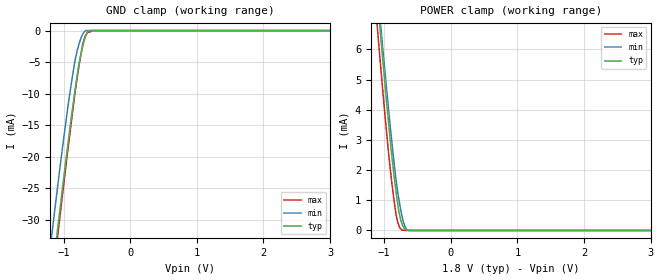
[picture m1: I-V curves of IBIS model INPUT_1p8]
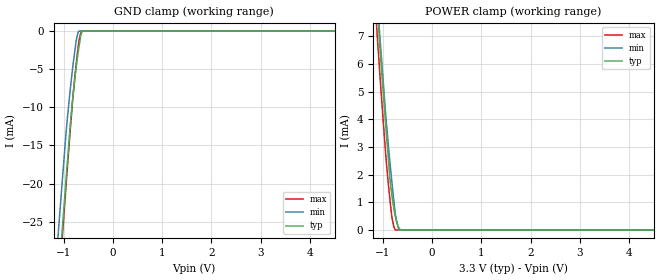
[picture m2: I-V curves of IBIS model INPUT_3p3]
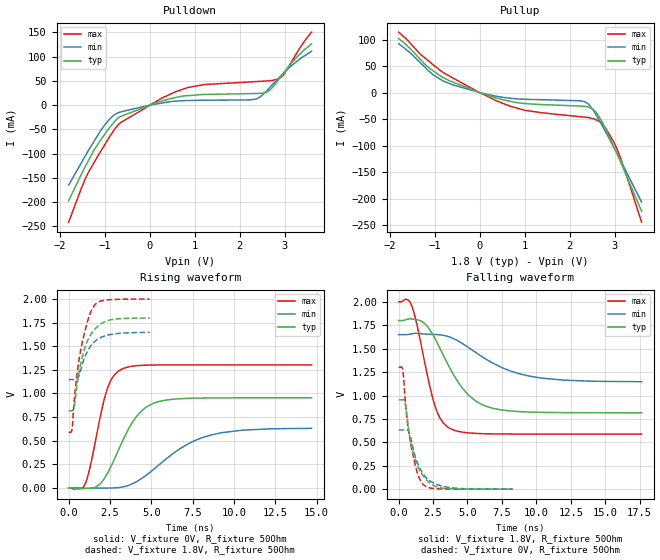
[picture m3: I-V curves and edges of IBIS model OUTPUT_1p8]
|Texas Instruments Incorporated
|12-Bit, Nanopower, 4-Wire
|   Micro TOUCH SCREEN CONTROLLER with I2C Interface
| Marketing part#   Digital Voltage Range   Package-type   #pins
|TSC2017IYZGT   1.6V - 3.6V   3X4 Array, WCSP   12-pins
|TSC2017IYZGR   1.6V - 3.6V   3X4 Array, WCSP   12-pins
[IBIS Ver]   4.0
[File name]   tsc2017.ibs
|SIMDE Ver   V2.0 - 201002 - RHL4 - Build 372
[File Rev]   1.0
[Date]   02/18/2011
[Source]   Texas Instruments Incorporated.
   Analog-eLab, HPA
   12500 TI Blvd
   Dallas, TX -75243
   For Support e-mail: elab_ibis@list.ti.com
[Notes]   Revision History:
   1.0: 02/18/2011
   - Initial version of the model
   - Model generated from simulations in TISPICE
   - Model matched to SPICE simulation
   - C_comp although listed in numerical order of value are
   obtained from varying PVT conditions. For PVT conditions for
   each specific value refer the buffer description under
   respective [Model]. IBIS model user is responsible for using
   appropriate C_comp to simulate for Signal Integrity.
   1.1: 03/17/2011
   - Removed 50 ohm loads rising waveform and falling waveform data
   for I2C_fast_mode_1p8, I2C_fast_mode_3p3,
   I2C_high_mode_1p8, and I2C_high_mode_3p3 buffers.
[Disclaimer]
 This product is designed as an aid for customers of Texas Instruments.
 No warranties, either expressed or implied, with respect to this third
 party software (if any) or with respect to its fitness for any
 particular purpose is claimed by Texas Instruments or the author. The
 software (if any) is provided solely on an "as is" basis. The entire
 risk as to its quality and performance is with the customer
[Copyright] (C) Copyright 2011 Texas Instruments Incorporated.
   All rights reserved.
|   TSC2017
[Component]   tsc2017yzg
[Manufacturer] TI
[Package]   |12 WCSP -  YZG package
| variable   typ   min   max
R_pkg   5.30000E-02   1.00000E-03   1.81000E-01
L_pkg   5.36400E-01nH 1.07000E-01nH 1.65500E+00nH
C_pkg   7.09400E-01pF 4.30000E-01pF 1.27400E+00pF
[Pin] signal_name  model_name  R_pin  L_pin C_pin
A1   AUX   TERM   0.007   0.211nH   0.551pF
A2   VDD_REF   POWER   0.004   0.165nH   0.711pF
A3   XP   TERM   0.011   0.249nH   0.568pF
B1   _PINTDAV   OUTPUT   0.181   1.655nH   1.274pF
B2   A0   INPUT   0.042   0.651nH   0.989pF
B3   YP   TERM   0.005   0.189nH   0.554pF
C1   SDA   I2C   0.001   0.107nH   0.430pF
C2   _RESET   INPUT   0.101   0.728nH   0.719pF
C3   XN   TERM   0.007   0.190nH   0.517pF
D1   SCL   I2C   0.163   1.109nH   0.887pF
D2   GND   GND   0.010   0.142nH   0.687pF
D3   YN   TERM   0.012   0.275nH   0.605pF
|   Model Selectors
[Model Selector] INPUT
INPUT_1p8   1.8V digital input
INPUT_3p3   3.3V digital input
|NOTES   Model INPUT split into two Models INPUT_1p6, INPUT_1p8 and
|   INPUT_3p3 to accomodate voltage range of 1.6 V - 3.6V
|   INPUT_1p8 operates in voltage range of 1.65 - 1.8 - 2.0
|   INPUT_3p3 operates in voltage range of 3.0 - 3.3 - 3.6
|   The min pin frequency for Model INPUT is 400 KHz
|   This is referenced with datasheet
[Model Selector] I2C
I2C_fast_mode_1p8   1.8V digital open drain io
I2C_fast_mode_3p3   3.3V digital open drain io
I2C_high_mode_1p8   1.8V digital open drain io
I2C_high_mode_3p3   3.3V digital open drain io
|NOTES   Model I2C split into four Models
|   I2C_fast_mode_1p8, I2C_fast_mode_3p3,
|   I2C_high_mode_1p8 and I2C_high_mode_3p3 to accomodate
|   voltage range of 1.6 V - 3.6V and high speed and fast speed
|   modes. I2C_fast_mode operates at 400 KHz and I2C_high_mode
|   operates at 3.4 MHz. This is referenced with datasheet
[Model Selector] OUTPUT
OUTPUT_1p8   1.8V digital output
OUTPUT_3p3   3.3V digital output
|NOTES   Model OUTPUT split into two Models OUTPUT_1p8 and
|   OUTPUT_3p3 to accomodate voltage range of 1.6 V - 3.6V
|   OUTPUT_1p8 operates in voltage range of 1.65 - 1.8 - 2.0
|   OUTPUT_3p3 operates in voltage range of 3.0 - 3.3 - 3.6
|   The min pin frequency for Model OUTPUT is 400 KHz
|   This is referenced with datasheet
[Model Selector] TERM
TERM_1p8  1.8V nominal termination
TERM_3p3  3.3V nominal termination
|   TERM Models
[Model] TERM_1p8
Model_type Terminator
C_comp   1.0e-20F  1.0e-20F  1.0e-20F
|   typ   min   max
[Voltage Range]   1.8V   1.65V   2.0V
[POWER Clamp Reference]   1.8V   1.65V   2.0V
[GND Clamp Reference]   0V   0V   0V
|Ambient Temperature   25   85   -40
|Junction Temperature
[Temperature Range]   25   85   -40
[Model] TERM_3p3
Model_type Terminator
C_comp   1.0e-20F  1.0e-20F  1.0e-20F
|   typ   min   max
[Voltage Range]   3.3V   3.0V   3.6V
[POWER Clamp Reference]   3.3V   3.0V   3.6V
[GND Clamp Reference]   0V   0V   0V
|Ambient Temperature   25   85   -40
|Junction Temperature
[Temperature Range]   25   85   -40
| Models and submodels in the file (10): INPUT_1p8 (Input), INPUT_3p3 (Input), OUTPUT_1p8 (Output), OUTPUT_3p3 (Output), I2C_fast_mode_1p8 (I/O_open_drain), I2C_fast_mode_3p3 (I/O_open_drain), I2C_high_mode_1p8 (I/O_open_drain), I2C_high_mode_3p3 (I/O_open_drain), TERM_1p8 (Terminator), TERM_3p3 (Terminator)
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|   input_1p8 Model
[Model]   INPUT_1p8
Model_type   Input
Vinl = 0.54
Vinh = 1.26
|   typ   min   max
|   (nom PVT)   (Fast PVT)   (slow PVT)
|Average
C_comp   9.562e-12   9.071e-12   9.997e-12
|C_comp from frequency method(F=3.4MHz)
| Where nom  PVT is Nominal Process, 1.8V, 25C
|   Fast PVT is Strong Process,  2V, -40C
|   Slow PVT is Weak Process,   1.65V, 85C
[Model Spec]
Vinl   0.54   0.495   0.6
Vinh   1.26   1.155   1.4
[Voltage Range]   1.8   1.65   2
|Ambient Temperature   25   85   -40
|Junction Temperature
[Temperature Range]   25   85   -40
[Power Clamp Reference]   1.8   1.65   2
[GND Clamp Reference]   0   0   0
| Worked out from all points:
|   GND clamp passes 1 mA (typ) near -0.67 V on its own axis
|   POWER clamp passes 1 mA (typ) near -0.80 V on its own axis
[GND Clamp]
|   Voltage   I(typ)   I(min)   I(max)
-1.8V     -97.74mA   -89.52mA   -99.7mA
-1.216V   -43.04mA   -35.82mA   -44.31mA
-1.135V   -35.66mA   -28.69mA   -36.85mA
-1.086V   -31.2mA    -24.48mA   -32.33mA
-1.048V   -27.78mA   -21.18mA   -28.86mA
-938.7mV  -18.34mA   -12.35mA   -19.16mA
-829.8mV  -9.61mA    -4.831mA   -10.01mA
-779.4mV  -5.962mA   -2.543mA   -6.355mA
-714mV    -2.549mA   -619.2uA   -2.193mA
-673.1mV  -933.1uA   -19.37uA   -877.4uA
-621mV    0A         0A         -230.3uA
3.6V      0A         0A         0A
[POWER Clamp]
|   Voltage   I(typ)   I(min)   I(max)
-1.8V     26.45mA    26.22mA    26.14mA
-1.136V   8.566mA    8.855mA    7.605mA
-1.074V   6.979mA    7.313mA    5.97mA
-1.038V   6.072mA    6.436mA    5.035mA
-932mV    3.516mA    3.939mA    2.501mA
-882mV    2.391mA    2.86mA     1.516mA
-820mV    1.249mA    1.644mA    496.9uA
-781.2mV  633.6uA    1.059mA    174.8uA
-742mV    277.5uA    570.3uA    22.96uA
-687.9mV  51.63uA    132.1uA    0A
-646.6mV  1.062uA    10.03uA    0A
3.6V      0A         0A         0A
|   input_3p3 Model
[Model]   INPUT_3p3
Model_type   Input
Vinl = 0.99
Vinh = 2.31
|   typ   min   max
|   (nom PVT)   (Fast PVT)   (slow PVT)
|Average
C_comp   8.331e-12   7.932e-12   8.729e-12
|C_comp from frequency method(F=3.4MHz)
| Where nom  PVT is Nominal Process, 3.3V, 25C
|   Fast PVT is Strong Process,  3.6V, -40C
|   Slow PVT is Weak Process,   3V, 85C
[Model Spec]
Vinl   0.99   0.9   1.08
Vinh   2.31   2.1   2.52
[Voltage Range]   3.3   3   3.6
|Ambient Temperature   25   85   -40
|Junction Temperature
[Temperature Range]   25   85   -40
[Power Clamp Reference]   3.3   3   3.6
[GND Clamp Reference]   0   0   0
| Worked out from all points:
|   GND clamp passes 1 mA (typ) near -0.66 V on its own axis
|   POWER clamp passes 1 mA (typ) near -0.80 V on its own axis
[GND Clamp]
|   Voltage   I(typ)   I(min)   I(max)
-3.3V     -241.1mA   -231.5mA   -244.6mA
-1.104V   -32.85mA   -26.03mA   -33.97mA
-1.053V   -28.23mA   -21.71mA   -29.31mA
-1.016V   -25.06mA   -18.68mA   -26.07mA
-939mV    -18.45mA   -12.41mA   -19.18mA
-851.4mV  -11.2mA    -6.805mA   -11.79mA
-816mV    -8.891mA   -4.739mA   -8.9mA
-747mV    -4.835mA   -1.28mA    -4.399mA
-690mV    -2.104mA   0A         -1.276mA
-653.4mV  -561.9uA   0A         -288uA
-621mV    0A         0A         0A
6.6V      0A         0A         0A
[POWER Clamp]
|   Voltage   I(typ)   I(min)   I(max)
-3.3V     67.48mA    66.37mA    68.35mA
-1.122V   8.218mA    8.51mA     7.239mA
-1.061V   6.644mA    7.01mA     5.622mA
-942mV    3.797mA    4.163mA    2.723mA
-888mV    2.58mA     3.058mA    1.647mA
-851.4mV  1.764mA    2.36mA     1.017mA
-816mV    1.25mA     1.716mA    455.8uA
-751.2mV  537.4uA    640.5uA    73.8nA
-723mV    314.5uA    341.8uA    0A
-669.9mV  64.54uA    0A         0A
-621.6mV  0A         0A         0A
6.6V      0A         0A         0A
|   output_1p8 Model
[Model]   OUTPUT_1p8
Model_type   Output
Polarity   Non-Inverting
Enable   Active-Low
Vmeas = 0.9
Vref = 0.9
Cref = 15pF
Rref = 50
|   typ   min   max
|   (nom PVT)   (Fast PVT)   (slow PVT)
|Average
C_comp   1.623e-11   1.530e-11   1.723e-11
|ON state : BUFFER OUTPUT TURNED HIGH
|C_comp   1.504e-11   1.382e-11   1.648e-11
|OFF state: BUFFER OUTPUT TURNED LOW
|C_comp   1.741e-11   1.677e-11   1.797e-11
|C_comp from frequency method(F=3.4MHz)
| Where nom  PVT is Nominal Process, 1.8V, 25C
|   Fast PVT is Strong Process,  2V, -40C
|   Slow PVT is Weak Process,   1.65V, 85C
[Voltage Range]   1.8   1.65   2
|Ambient Temperature   25   85   -40
|Junction Temperature
[Temperature Range]   25   85   -40
[Pullup Reference]   1.8   1.65   2
[Pulldown Reference]   0   0   0
[Power Clamp Reference]   1.8   1.65   2
[GND Clamp Reference]   0   0   0
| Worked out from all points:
|   slope of the pulldown table from 0 to 0.27 V, typ, clamps not added: 32.4 ohm
|   slope of the pullup table from 0 to 0.27 V, typ, clamps not added: 35.8 ohm
|   falling waveform, V_fixture 1.8V, R_fixture 50Ohm: 20-80 % time 2.37ns typ, 3.73ns min, 1.3ns max; typ from 1.8 V to 0.816 V
|   rising waveform, V_fixture 0V, R_fixture 50Ohm: 20-80 % time 1.68ns typ, 3.06ns min, 978ps max; typ from 0 V to 0.954 V
|   rising waveform, V_fixture 1.8V, R_fixture 50Ohm: 20-80 % time 816ps typ, 826ps min, 763ps max; typ from 0.816 V to 1.8 V
|   falling waveform, V_fixture 0V, R_fixture 50Ohm: 20-80 % time 937ps typ, 1.03ns min, 770ps max; typ from 0.954 V to 0 V
[Pulldown]
|   Voltage   I(typ)   I(min)   I(max)
-1.8V     -197mA     -164.9mA   -241.6mA
-1.366V   -115.3mA   -94.35mA   -139.7mA
-909mV    -48.61mA   -30.78mA   -68.04mA
-658mV    -23.84mA   -14.4mA    -36.91mA
280mV     8.607mA    4.451mA    14.94mA
842mV     19.73mA    9.519mA    36.23mA
2.221V    23.86mA    10.83mA    47.87mA
2.432V    24.3mA     15.44mA    48.99mA
2.594V    26.87mA    28.95mA    49.84mA
2.938V    61.39mA    62.64mA    58.87mA
3.278V    99.9mA     90.73mA    108.8mA
3.6V      126.5mA    111.2mA    150.8mA
[Pullup]
|   Voltage   I(typ)   I(min)   I(max)
-1.8V     101.8mA    91.99mA    114mA
-1.193V   51.39mA    45.91mA    63.68mA
-810mV    28.31mA    21.74mA    37.82mA
342mV     -9.558mA   -6.441mA   -14.24mA
1.03V     -20.83mA   -12.63mA   -33.68mA
2.327V    -25.94mA   -16.91mA   -46.26mA
2.527V    -32.07mA   -33.7mA    -49.43mA
2.668V    -47.21mA   -53.65mA   -54.9mA
2.818V    -71.33mA   -76.76mA   -69.56mA
3.052V    -115.3mA   -114.6mA   -105.8mA
3.25V     -153.9mA   -147.7mA   -152.4mA
3.6V      -223.7mA   -206.4mA   -244.3mA
[Ramp]
R_load = 50
|   typ   min   max
dV/dt_r   0.572113/1.68018e-09   0.379155/3.06207e-09   0.781483/9.76981e-10
dV/dt_f   0.590487/2.36674e-09   0.301912/3.72302e-09   0.846765/1.29693e-09
[Falling Waveform]
V_fixture = 1.8V
V_fixture_min = 1.65V
V_fixture_max = 2V
R_fixture = 50Ohm
|   Time   V(typ)   V(min)   V(max)
0s        1.8V       1.65V      2V
925ps     1.817V     1.658V     1.968V
1.9ns     1.767V     1.656V     1.347V
2.6ns     1.619V     1.652V     907.8mV
3.1ns     1.474V     1.646V     737mV
3.65ns    1.313V     1.628V     655.1mV
5.15ns    994.5mV    1.505V     600.1mV
6.825ns   864.2mV    1.347V     590.4mV
10.4ns    820mV      1.186V     588.7mV
17.65ns   815.9mV    1.148V     588.7mV
[Rising Waveform]
V_fixture = 0V
V_fixture_min = 0V
V_fixture_max = 0V
R_fixture = 50Ohm
|   Time   V(typ)   V(min)   V(max)
0s        517.7pV    1.503nV    385.9pV
1ns       -6.01mV    -5.851mV   43.03mV
1.675ns   11.84mV    -3.376mV   545mV
2.325ns   146.9mV    -2.441mV   1.042V
2.675ns   268mV      -1.458mV   1.174V
3.2ns     473.1mV    6.896mV    1.256V
4.325ns   799.7mV    87.88mV    1.297V
5.525ns   917.1mV    251.8mV    1.302V
8.625ns   952.2mV    559.9mV    1.302V
14.7ns    953.5mV    630.6mV    1.302V
[Rising Waveform]
V_fixture = 1.8V
V_fixture_min = 1.65V
V_fixture_max = 2V
R_fixture = 50Ohm
|   Time   V(typ)   V(min)   V(max)
0s        815.8mV    1.146V     588.7mV
200ps     815.5mV    1.147V     616.5mV
325ps     847mV      1.146V     910.1mV
425ps     972.1mV    1.145V     1.084V
550ps     1.144V     1.162V     1.262V
750ps     1.334V     1.258V     1.479V
1.15ns    1.561V     1.451V     1.769V
1.475ns   1.658V     1.533V     1.912V
2.525ns   1.779V     1.624V     1.994V
4.9ns     1.799V     1.647V     2V
[Falling Waveform]
|Gnd
V_fixture = 0V
V_fixture_min = 0V
V_fixture_max = 0V
R_fixture = 50Ohm
|   Time   V(typ)   V(min)   V(max)
0s        953.5mV    632mV      1.302V
300ps     954.4mV    631.8mV    1.271V
450ps     932.4mV    632.6mV    1V
600ps     788.4mV    633.8mV    761.1mV
775ps     587.8mV    600.5mV    569.6mV
975ps     433mV      487.3mV    409.6mV
1.375ns   244mV      276mV      166.5mV
1.775ns   142.6mV    162.5mV    52.32mV
3.125ns   12.78mV    34.05mV    2.859mV
8.275ns   72.01uV    343.7uV    11.7uV
